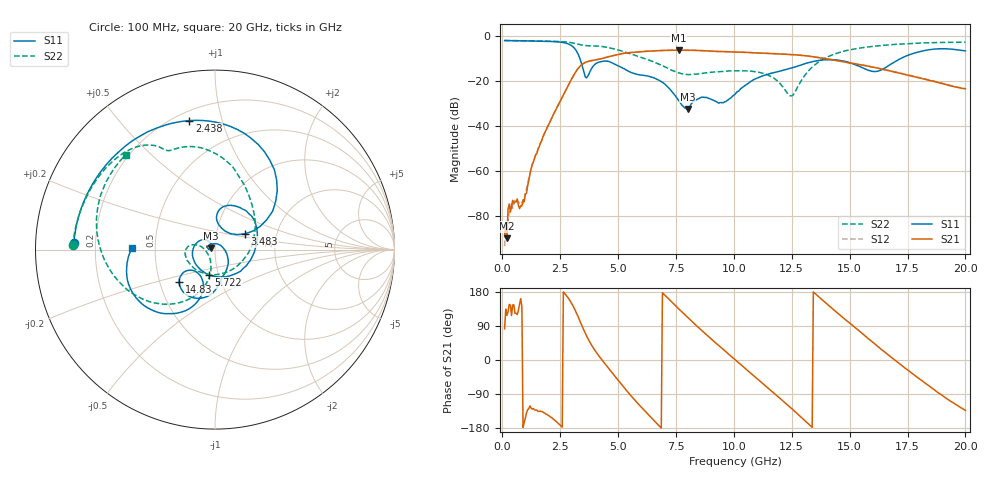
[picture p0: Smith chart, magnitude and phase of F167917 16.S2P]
!  2-Port S-parameters saved by WinCal
! VAR MeasName=S-Parameters (CALIBRATED_DATA) read from VNA (N5242A)
! VAR MeasDate=2016-11-22 9:00:27
! VAR NAME=F167917 16
! VAR FILENAME=F167917 16.S2P
! VAR DATE=2016-11-22 9:00:27
! VAR PHYS_PORTS=1,2
# Hz S DB R 50
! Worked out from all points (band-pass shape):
!   401 points, 100 MHz to 20 GHz, reference 50 ohm
!   highest |S21| = -6.34 dB at 7.612 GHz (marker M1); lowest = -89.7 dB at 199.5 MHz (marker M2)
!   |S21| within 3 dB of the highest: 4.542 GHz to 13.47 GHz (8.931 GHz wide, 99.1 % of centre)
!   lowest |S11| = -32.4 dB at 8.01 GHz (marker M3), VSWR 1.05, Z = 47.8 + j0.758 ohm
!   |S11| at or under -10 dB: 3.349 GHz to 17.21 GHz (13.87 GHz wide, 135 % of centre)
!   |S22| runs from -26.6 to -2.0 dB; largest |S21 - S12| = 0.0043
!   S11 on the Smith chart (normalised r, x): 100 MHz: 0.12, +0.02; 2.438 GHz: 0.25, +0.79; 3.483 GHz: 1.37, +0.25; 5.722 GHz: 0.90, -0.26; 14.83 GHz: 0.63, -0.25; 20 GHz: 0.37, +0.01
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1e8  -2.08 177.3  -88.52 82.5  -93.27 -166.0  -2.03 178.3
1.995e8  -2.09 174.7  -89.70 117.9  -85.58 65.2  -2.04 176.6
8.4625e8  -2.19 157.4  -75.48 140.3  -73.84 157.8  -2.14 166.2
1.34375e9  -2.28 143.3  -55.90 -128.0  -55.80 -130.7  -2.22 158.2
2.43825e9  -2.70 101.3  -30.24 -168.2  -30.23 -168.8  -2.49 137.9
3.085e9  -5.13 53.3  -17.46 139.4  -17.48 139.1  -3.21 122.5
3.43325e9  -12.66 26.1  -12.74 91.2  -12.74 91.2  -4.09 116.8
3.483e9  -14.54 27.8  -12.38 84.3  -12.36 84.2  -4.17 116.4
3.682e9  -18.02 73.2  -11.42 58.3  -11.40 58.2  -4.35 114.3
4.5775e9  -11.25 37.0  -9.25 -21.2  -9.25 -21.4  -5.20 92.8
5.72175e9  -16.81 -103.6  -7.23 -105.9  -7.21 -105.9  -8.58 61.4
6.7665e9  -19.66 154.7  -6.53 -173.3  -6.53 -173.5  -12.56 21.0
7.61225e9  -28.65 127.8  -6.34 135.4  -6.37 135.3  -16.36 -39.7
8.01025e9  -32.44 160.6  -6.39 112.5  -6.39 112.4  -17.16 -75.7
1.005e10  -25.92 2.4  -7.13 0.9  -7.15 1.1  -15.54 -165.9
1.1443e10  -17.08 -66.3  -7.80 -72.2  -7.74 -71.9  -17.24 169.7
1.248775e10  -14.28 -84.5  -8.30 -127.7  -8.29 -127.7  -26.62 -145.8
1.338325e10  -11.46 -100.4  -9.18 -177.7  -9.13 -177.5  -13.84 -105.2
1.4826e10  -11.36 -137.7  -11.70 106.1  -11.61 106.2  -6.59 -141.8
1.67165e10  -12.98 -106.9  -15.46 11.2  -15.41 11.7  -3.96 -179.0
1.8209e10  -6.54 -131.9  -19.13 -58.7  -18.91 -58.7  -3.11 157.7
2e10  -6.67 179.1  -23.48 -133.1  -23.35 -133.7  -2.80 133.3
